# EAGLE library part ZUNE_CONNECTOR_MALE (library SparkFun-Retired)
Male connector for the Zune media player. UNPROVEN FOOTPRINT! This connector must be used only with a 1.2mm PCB thickness.
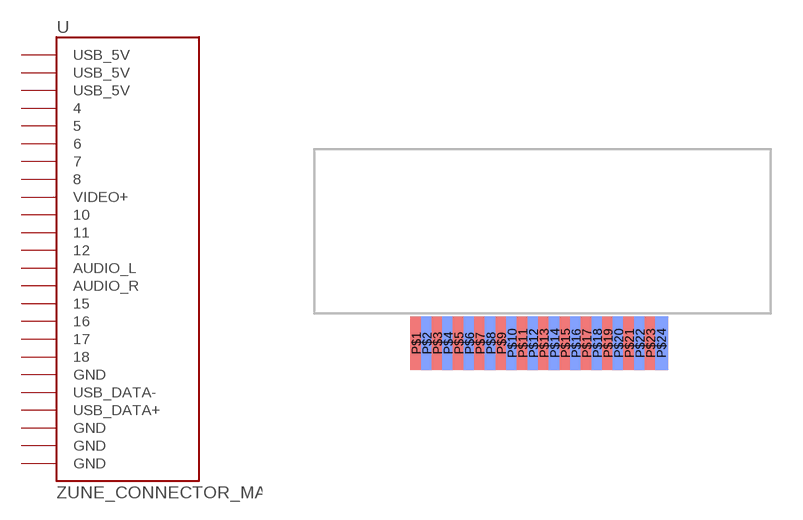
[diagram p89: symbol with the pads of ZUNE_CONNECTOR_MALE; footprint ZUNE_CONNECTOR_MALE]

Designator prefix -

## ZUNE_CONNECTOR_MALE  [ZUNE_CONNECTOR_MALE]
P$1  USB_5V
P$2  USB_5V
P$3  USB_5V
P$4  4
P$5  5
P$6  6
P$7  7
P$8  8
P$9  VIDEO+
P$10  10
P$11  11
P$12  12
P$13  AUDIO_L
P$14  AUDIO_R
P$15  15
P$16  16
P$17  17
P$18  18
P$19  GND
P$20  USB_DATA-
P$21  USB_DATA+
P$22  GND
P$23  GND
P$24  GND

## Footprint ZUNE_CONNECTOR_MALE (pad centres in mm)
smd 0.6 x 2.5: P$1 0,0; P$3 1,0; P$5 2,0; P$7 3,0; P$9 4,0; P$11 5,0; P$13 6,0; P$15 7,0; P$17 8,0; P$19 9,0; P$21 10,0; P$23 11,0
smd 0.6 x 2.5 bottom: P$2 0.5,0; P$4 1.5,0; P$6 2.5,0; P$8 3.5,0; P$10 4.5,0; P$12 5.5,0; P$14 6.5,0; P$16 7.5,0; P$18 8.5,0; P$20 9.5,0; P$22 10.5,0; P$24 11.5,0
